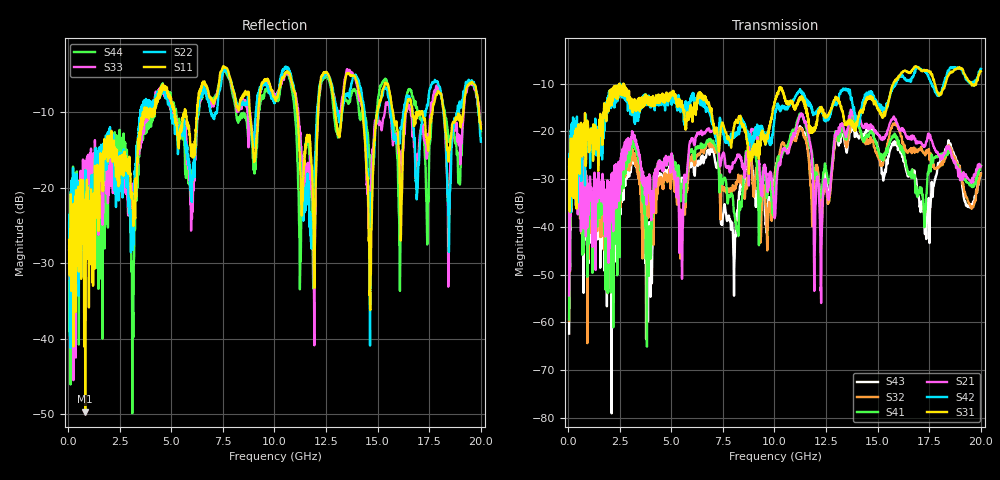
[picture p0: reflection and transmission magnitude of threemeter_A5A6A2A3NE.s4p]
! FILE: D:\iPass\iPassCable1005\iPassCable\SOLT_cal\threemeter_A5A6A2A3NE.s4p
# MHz S MA R 50.00
! FREQ  S11  S12  S13  S14
!  S21  S22  S23  S24
!  S31  S32  S33  S34
!  S41  S42  S43  S44
!  MAG  ANG  MAG  ANG  MAG  ANG  MAG  ANG
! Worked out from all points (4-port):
!   1996 points, 50 MHz to 20 GHz, reference 50 ohm
!   strongest paths, dB at 50 MHz, 5.04 GHz, 10.03 GHz, 15.02 GHz, 20 GHz:
!     S31: -28.8, -11.9, -13.6, -15.5, -7.5
!     S42: -27.5, -13.1, -15.7, -14.4, -6.9
!     S21: -54.4, -25.3, -37.8, -20.6, -27.3
!     S41: -59.4, -25.1, -31.5, -23.7, -27.1
!     S32: -59.7, -28.2, -29.2, -24.8, -28.9
!     S43: -62.3, -27.1, -28.4, -23.4, -28.8
!   lowest |S11| = -49.7 dB at 830 MHz (marker M1), VSWR 1.01, Z = 50.3 - j0.127 ohm
!   |S11| at or under -10 dB: start of sweep to 3.659 GHz; 11.1 GHz to 12.11 GHz (1.006 GHz wide, 8.67 % of centre); 18.21 GHz to 19.15 GHz (941.4 MHz wide, 5.04 % of centre)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
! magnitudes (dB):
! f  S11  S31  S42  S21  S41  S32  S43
! 50 MHz  -26.9  -28.8  -27.5  -54.4  -59.4  -59.7  -62.3
! 250 MHz  -22.7  -21.5  -18.3  -27.0  -26.8  -27.6  -27.3
! 830 MHz  -49.7  -19.1  -27.2  -29.3  -30.9  -29.7  -30.6
! 7.56 GHz  -4.0  -19.2  -21.6  -24.7  -29.7  -31.7  -35.6
! 13.86 GHz  -5.2  -19.6  -15.3  -17.2  -17.2  -18.4  -19.4
! 14.64 GHz  -36.2  -12.6  -12.1  -19.3  -20.0  -21.5  -19.0
! 20 GHz  -12.2  -7.5  -6.9  -27.3  -27.1  -28.9  -28.8
